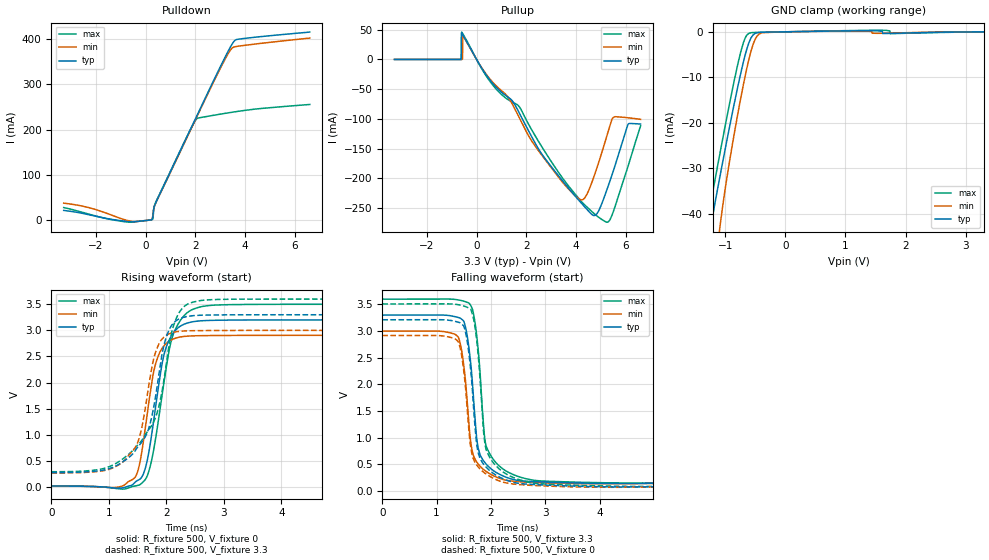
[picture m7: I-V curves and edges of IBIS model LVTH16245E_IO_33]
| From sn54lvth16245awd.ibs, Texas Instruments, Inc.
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[Model]   LVTH16245E_IO_33
Model_type  I/O
Vinl=1.05
Vinh=2.34
Enable   Active-Low
Vref =   0
Rref =   500
Cref =   50p
Vmeas =   1.5
| variable   typ   min   max
C_comp   3.26pF   2.49pF   3.81pF
| C_pullup   4.38pF   0.46pF   12.23pF
| C_pulldown   3.27pF   2.52pF   3.91pF
| C_tri-state   3.26pF   2.49pF   3.81pF
[Temperature Range]   40   100   -40
| Ambient temperature   25   85   -40
[Voltage range]   3.3   3   3.6
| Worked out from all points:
|   slope of the pulldown table from 0 to 0.495 V, typ, clamps not added: 9.89 ohm
|   slope of the pullup table from 0 to 0.495 V, typ, clamps not added: 15.3 ohm
|   GND clamp passes 1 mA (typ) near -0.55 V on its own axis
|   rising waveform, R_fixture 500, V_fixture 0: 20-80 % time 273ps typ, 245ps min, 307ps max; typ from 0.018 V to 3.2 V
|   falling waveform, R_fixture 500, V_fixture 3.3: 20-80 % time 163ps typ, 161ps min, 160ps max; typ from 3.3 V to 0.226 V
|   rising waveform, R_fixture 500, V_fixture 3.3: 20-80 % time 368ps typ, 293ps min, 479ps max; typ from 0.278 V to 3.3 V
|   falling waveform, R_fixture 500, V_fixture 0: 20-80 % time 184ps typ, 184ps min, 185ps max; typ from 3.21 V to 0.035 V
[GND Clamp]
| LVTH16245E_IO_33
|   Voltage   I(typ)   I(min)   I(max)
-3.3V     -660.6mA   -694.1mA   -619.5mA
-1.315V   -49.89mA   -78.93mA   -43.2mA
-1.295V   -47.94mA   -74.56mA   -41.74mA
-1.23V    -42.35mA   -62.17mA   -37.03mA
-1.085V   -31.78mA   -42.85mA   -26.71mA
-925mV    -20.85mA   -28.41mA   -15.72mA
-740mV    -9.123mA   -14.59mA   -4.435mA
-665mV    -5.024mA   -9.624mA   -1.319mA
-605mV    -2.415mA   -6.085mA   -341.7uA
-505mV    -375.1uA   -1.783mA   -148.7uA
-385mV    -98.12uA   -193uA     -112uA
3.3V      167pA      22.82nA    15.75pA
[Pulldown]
| LVTH16245E_IO_33
|   Voltage   I(typ)   I(min)   I(max)
-3.3V     22.21mA    38.12mA    28.43mA
-2.215V   11.78mA    27.17mA    12.84mA
-895mV    -1.372mA   2.37mA     -2.459mA
-445mV    -2.787mA   -2.502mA   -2.903mA
235mV     1.673mA    2.065mA    1.482mA
285mV     8.717mA    10.91mA    3.537mA
335mV     28.95mA    28.08mA    29.22mA
420mV     41.13mA    40.47mA    42.09mA
2.02V     226.1mA    224mA      221.8mA
3.18V     358.2mA    353.7mA    235.6mA
3.55V     394.2mA    381.9mA    238.9mA
6.6V      414.7mA    401.5mA    255.3mA
[Pullup]
| LVTH16245E_IO_33
|   Voltage   I(typ)   I(min)   I(max)
-3.3V     63.99uA    73.67uA    58.75uA
-625mV    43.57uA    54.62uA    43.48uA
-610mV    43.03mA    51.81uA    40.03uA
-595mV    44.87mA    49.11uA    46.07mA
-530mV    39.9mA     39.09mA    41.56mA
2.38V     -142.5mA   -147.2mA   -130.1mA
4.155V    -239mA     -235.6mA   -236.1mA
4.765V    -262.6mA   -192.2mA   -260.8mA
5.225V    -221.6mA   -131.2mA   -273.9mA
5.49V     -189.2mA   -98.07mA   -257.6mA
6.095V    -109.4mA   -98.21mA   -179.7mA
6.6V      -108.7mA   -100.8mA   -111.6mA
[Ramp]
| LVTH16245E_IO_33
| variable   typ   min   max
dV/dt_r   1.93/2.79E-10   1.75/2.55E-10   2.13/3.15E-10
dV/dt_f   1.90/1.83E-10   1.72/1.84E-10   2.08/1.79E-10
R_load = 500
[Rising Waveform]
| LVTH16245E_IO_33
R_fixture =   500
C_fixture =   0
L_fixture =   0
V_fixture =   0
V_fixture_min = 0
V_fixture_max = 0
|   Time   V(typ)   V(min)   V(max)
0s        18.23mV    18.9mV     16.74mV
1.27ns    -8.263mV   37.55mV    -38.2mV
1.49ns    119.7mV    260.9mV    26.75mV
1.63ns    343.3mV    1.099V     137.3mV
1.81ns    1.508V     2.347V     905.7mV
1.925ns   2.356V     2.654V     1.751V
2.025ns   2.758V     2.774V     2.469V
2.27ns    3.098V     2.878V     3.231V
2.705ns   3.189V     2.9V       3.471V
24.42ns   3.202V     2.906V     3.502V
[Falling Waveform]
| LVTH16245E_IO_33
R_fixture =   500
C_fixture =   0
L_fixture =   0
V_fixture =   3.3
V_fixture_min = 3
V_fixture_max = 3.6
|   Time   V(typ)   V(min)   V(max)
0s        3.3V       3V         3.6V
1.4ns     3.255V     2.885V     3.585V
1.505ns   3.172V     2.315V     3.559V
1.605ns   2.603V     1.135V     3.515V
1.75ns    893.8mV    524mV      2.807V
1.875ns   548.1mV    390.9mV    1.089V
1.915ns   497mV      360.8mV    830.1mV
2.23ns    275.2mV    210.1mV    403mV
2.8ns     171.5mV    153.9mV    196.3mV
24.42ns   225.6mV    221.7mV    239.7mV
[Rising Waveform]
| LVTH16245E_IO_33
R_fixture =   500
C_fixture =   0
L_fixture =   0
V_fixture =   3.3
V_fixture_min = 3
V_fixture_max = 3.6
|   Time   V(typ)   V(min)   V(max)
0s        277.8mV    267.7mV    294.3mV
1.045ns   366.4mV    355.4mV    407.5mV
1.275ns   507mV      510.7mV    564.8mV
1.54ns    815mV      984.6mV    847.7mV
1.725ns   1.246V     2.145V     1.145V
1.89ns    2.299V     2.78V      1.64V
2.01ns    2.908V     2.912V     2.439V
2.175ns   3.188V     2.975V     3.235V
2.62ns    3.291V     2.996V     3.575V
24.42ns   3.3V       3V         3.6V
[Falling Waveform]
| LVTH16245E_IO_33
R_fixture =   500
C_fixture =   0
L_fixture =   0
V_fixture =   0
V_fixture_min = 0
V_fixture_max = 0
|   Time   V(typ)   V(min)   V(max)
0s        3.212V     2.917V     3.51V
1.4ns     3.166V     2.798V     3.495V
1.52ns    3.029V     2.065V     3.464V
1.625ns   2.295V     834.7mV    3.414V
1.75ns    788.4mV    467.2mV    2.714V
1.865ns   498.6mV    348.9mV    1.099V
1.915ns   439.3mV    311.5mV    763.1mV
2.23ns    222.5mV    159.6mV    347.8mV
2.8ns     116.4mV    98.83mV    141.5mV
24.42ns   35.39mV    30.09mV    47.8mV
